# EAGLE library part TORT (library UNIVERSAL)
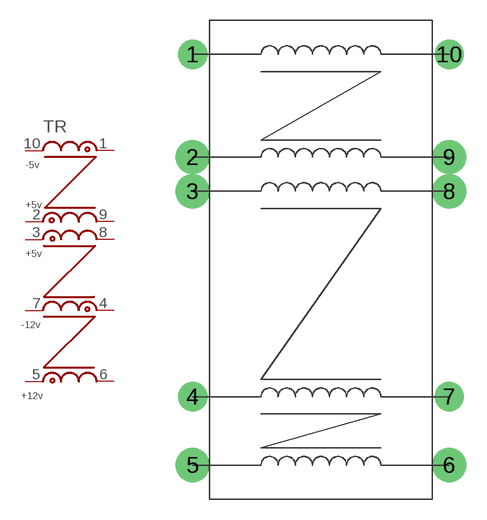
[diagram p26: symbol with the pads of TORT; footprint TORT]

Designator prefix TR

## TORT  [TORT]
1  1
2  2
3  3
4  4
5  5
6  6
7  7
8  8
9  9
10  10

## Footprint TORT (pad centres in mm)
drill 0.8 pad 2.184: 1 0,0; 4 0,-25.4; 7 19.05,-25.4; 10 19.05,0
drill 0.8 pad 2.54: 2 0,-7.62; 3 0,-10.16; 5 0,-30.48; 6 19.05,-30.48; 8 19.05,-10.16; 9 19.05,-7.62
